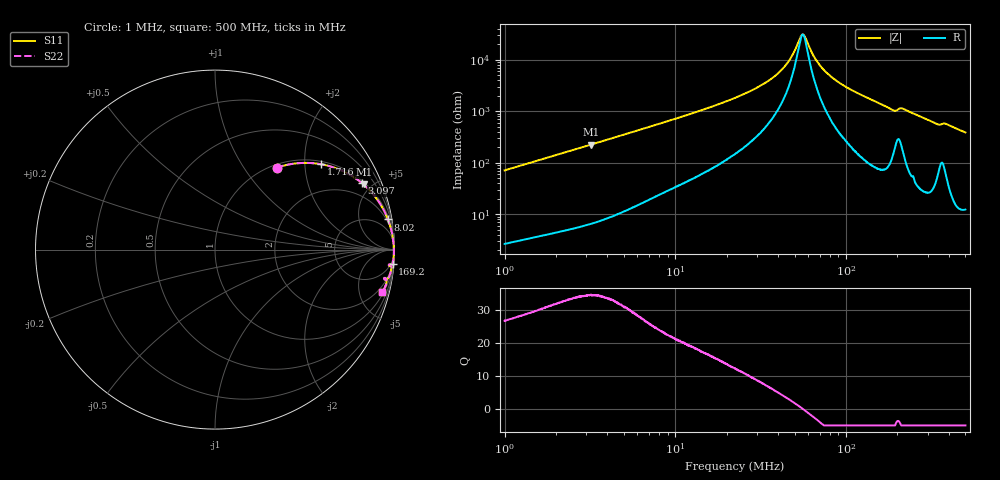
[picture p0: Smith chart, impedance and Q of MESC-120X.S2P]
!s-Parameter Generated by FASTRON Sdn. Bhd.
!FASTRON P/N : MESC-120X
!Keysight Technologies,E4991B,MY54100416,A.01.15
!Date: Mon Mar 16 11:09:04 2026
!Version  : Rev00 Mon Mar 16 11:09:04 2026
!Data & Calibration Information:
!PortZ  Port1:50+j0  Port2:50+j0
!When reading, reference impedance value at option line is always used.
! Remarks : This data is being provided solely for informational purposes.
!Freq	S11	S21	S12	S22
# Hz S dB R 50
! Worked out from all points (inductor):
!   1601 points, 1 MHz to 500 MHz, reference 50 ohm
!   read as one part in series: L = 11.3 uH near 1.032 MHz
!   highest Q = 34.4 at 3.207 MHz (marker M1), where L = 11.2 uH
!   self-resonance near 55.71 MHz
!   S11 on the Smith chart (normalised r, x): 1 MHz: 1.05, +1.43; 1.716 MHz: 1.08, +2.42; 3.097 MHz: 1.13, +4.35; 8.02 MHz: 1, +11; 169.2 MHz: 2, -25; 500 MHz: 1.25, -7.76
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1000000  -4.87 53.1  -1.94 -34.8  -1.94 -34.8  -4.87 53.1
1715825  -2.39 38.8  -4.06 -49.4  -4.06 -49.4  -2.39 38.8
2820919  -1.09 26.4  -7.03 -61.9  -7.03 -61.9  -1.09 26.4
3096529  -0.93 24.4  -7.68 -63.9  -7.68 -63.9  -0.93 24.4
3206689  -0.87 23.7  -7.93 -64.7  -7.93 -64.7  -0.87 23.7
7957584  -0.20 10.0  -15.22 -77.6  -15.22 -77.6  -0.20 10.0
8019641  -0.19 9.9  -15.29 -77.7  -15.29 -77.7  -0.19 9.9
2.236068e7  -0.05 3.1  -25.21 -82.2  -25.21 -82.2  -0.05 3.1
3.147229e7  -0.04 1.8  -29.89 -81.2  -29.89 -81.2  -0.04 1.8
4.004179e7  -0.03 1.0  -34.78 -77.4  -34.78 -77.4  -0.03 1.0
4.695421e7  -0.03 0.5  -40.20 -69.2  -40.20 -69.2  -0.03 0.5
5.527421e7  -0.03 0.0  -49.66 -9.1  -49.66 -9.1  -0.03 0.0
5.7687e7  -0.03 -0.1  -48.63 29.2  -48.63 29.2  -0.03 -0.1
6.307767e7  -0.03 -0.4  -42.74 63.9  -42.74 63.9  -0.03 -0.4
7.19828e7  -0.03 -0.8  -36.96 76.6  -36.96 76.6  -0.03 -0.8
8.707324e7  -0.03 -1.4  -32.02 81.8  -32.02 81.8  -0.03 -1.4
1.691754e8  -0.07 -4.5  -22.08 82.1  -22.08 82.1  -0.07 -4.5
1.77937e8  -0.09 -4.9  -21.36 80.7  -21.36 80.7  -0.09 -4.9
2.144052e8  -0.15 -4.9  -21.19 76.3  -21.19 76.3  -0.15 -4.9
3.377517e8  -0.25 -9.8  -15.38 75.7  -15.38 75.7  -0.25 -9.8
3.82452e8  -0.29 -9.7  -15.43 74.1  -15.43 74.1  -0.29 -9.7
5e8  -0.35 -14.3  -12.12 73.8  -12.12 73.8  -0.35 -14.3
